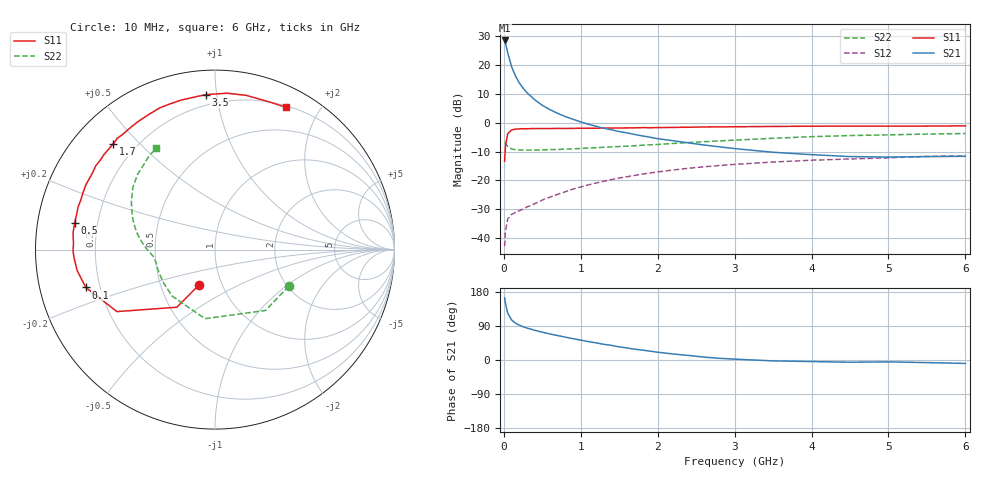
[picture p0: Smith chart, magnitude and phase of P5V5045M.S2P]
! SIEMENS Small Signal Semiconductors
! BFP183
! Si NPN RF Bipolar Junction Transistor in SOT143
! VCE = 0.5 V  IC = 45 mA
! Common Emitter S-Parameters:  March  1996
# GHz  S  MA  R  50
!  f  S11  S21  S12  S22
! GHz  MAG  ANG  MAG  ANG  MAG  ANG  MAG  ANG
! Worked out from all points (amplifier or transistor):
!   36 points, 10 MHz to 6 GHz, reference 50 ohm
!   highest |S21| = 28.6 dB at 10 MHz (marker M1)
!   |S21| within 3 dB of that: start of sweep to 39.02 MHz
!   unconditionally stable (mu >= 1): start of sweep to 26.31 MHz; 138 MHz to end of sweep
!   at 250 MHz: K = 1.45, MAG = 17.0 dB, |S12| = -30.0 dB
!   at 1.4 GHz: K = 2.12, MAG = 2.6 dB, |S12| = -19.7 dB
!   at 6 GHz: K = 1.48, MAG = -4.2 dB, |S12| = -11.4 dB
!   S11 on the Smith chart (normalised r, x): 10 MHz: 0.78, -0.32; 100 MHz: 0.15, -0.14; 500 MHz: 0.11, +0.09; 1.7 GHz: 0.12, +0.42; 3.5 GHz: 0.14, +0.93; 6 GHz: 0.22, +1.59
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0.01  0.2148 -114.2  26.96 164.4  0.0072 62.0  0.4587 -26.3
0.02  0.385 -123.5  24.62 150.7  0.0127 57.0  0.4407 -50.3
0.05  0.6464 -147.7  16.48 124.0  0.0213 42.0  0.3889 -98.2
0.1  0.7503 -163.7  9.502 105.9  0.0257 32.8  0.3524 -132.6
0.15  0.7769 -171.4  6.569 97.4  0.0277 33.2  0.3413 -147.3
0.2  0.786 -176.3  4.966 92.0  0.0297 36.8  0.3375 -155.1
0.25  0.7912 -179.6  3.994 87.7  0.0317 38.8  0.3369 -159.9
0.3  0.7889 177.8  3.349 84.4  0.0345 41.5  0.3363 -163.2
0.4  0.7964 173.3  2.522 78.5  0.0393 46.6  0.3364 -167.2
0.5  0.7959 169.4  2.014 73.5  0.0456 49.1  0.339 -169.9
0.6  0.7955 166.0  1.697 68.7  0.0513 51.7  0.3426 -171.8
0.7  0.7989 162.7  1.457 64.5  0.0572 53.3  0.3449 -173.2
0.9  0.8006 156.8  1.15 56.2  0.0707 54.5  0.3535 -175.3
1.1  0.804 150.5  0.943 48.5  0.0837 54.0  0.3642 -177.6
1.3  0.8121 144.9  0.804 41.4  0.0968 53.0  0.3756 -179.7
1.7  0.8176 133.8  0.628 28.6  0.122 49.2  0.3992 175.9
2.2  0.8322 121.2  0.489 15.9  0.1515 42.9  0.4382 169.1
2.8  0.8497 107.1  0.383 4.4  0.1812 34.6  0.4856 160.2
3.5  0.8652 93.5  0.308 -2.3  0.2084 25.7  0.5388 149.9
4.5  0.8768 78.6  0.259 -5.9  0.2353 13.9  0.6012 135.9
5.5  0.8784 68.1  0.259 -6.9  0.261 4.2  0.6379 125.2
6  0.8856 63.5  0.262 -9.0  0.2689 -0.9  0.6524 120.2
